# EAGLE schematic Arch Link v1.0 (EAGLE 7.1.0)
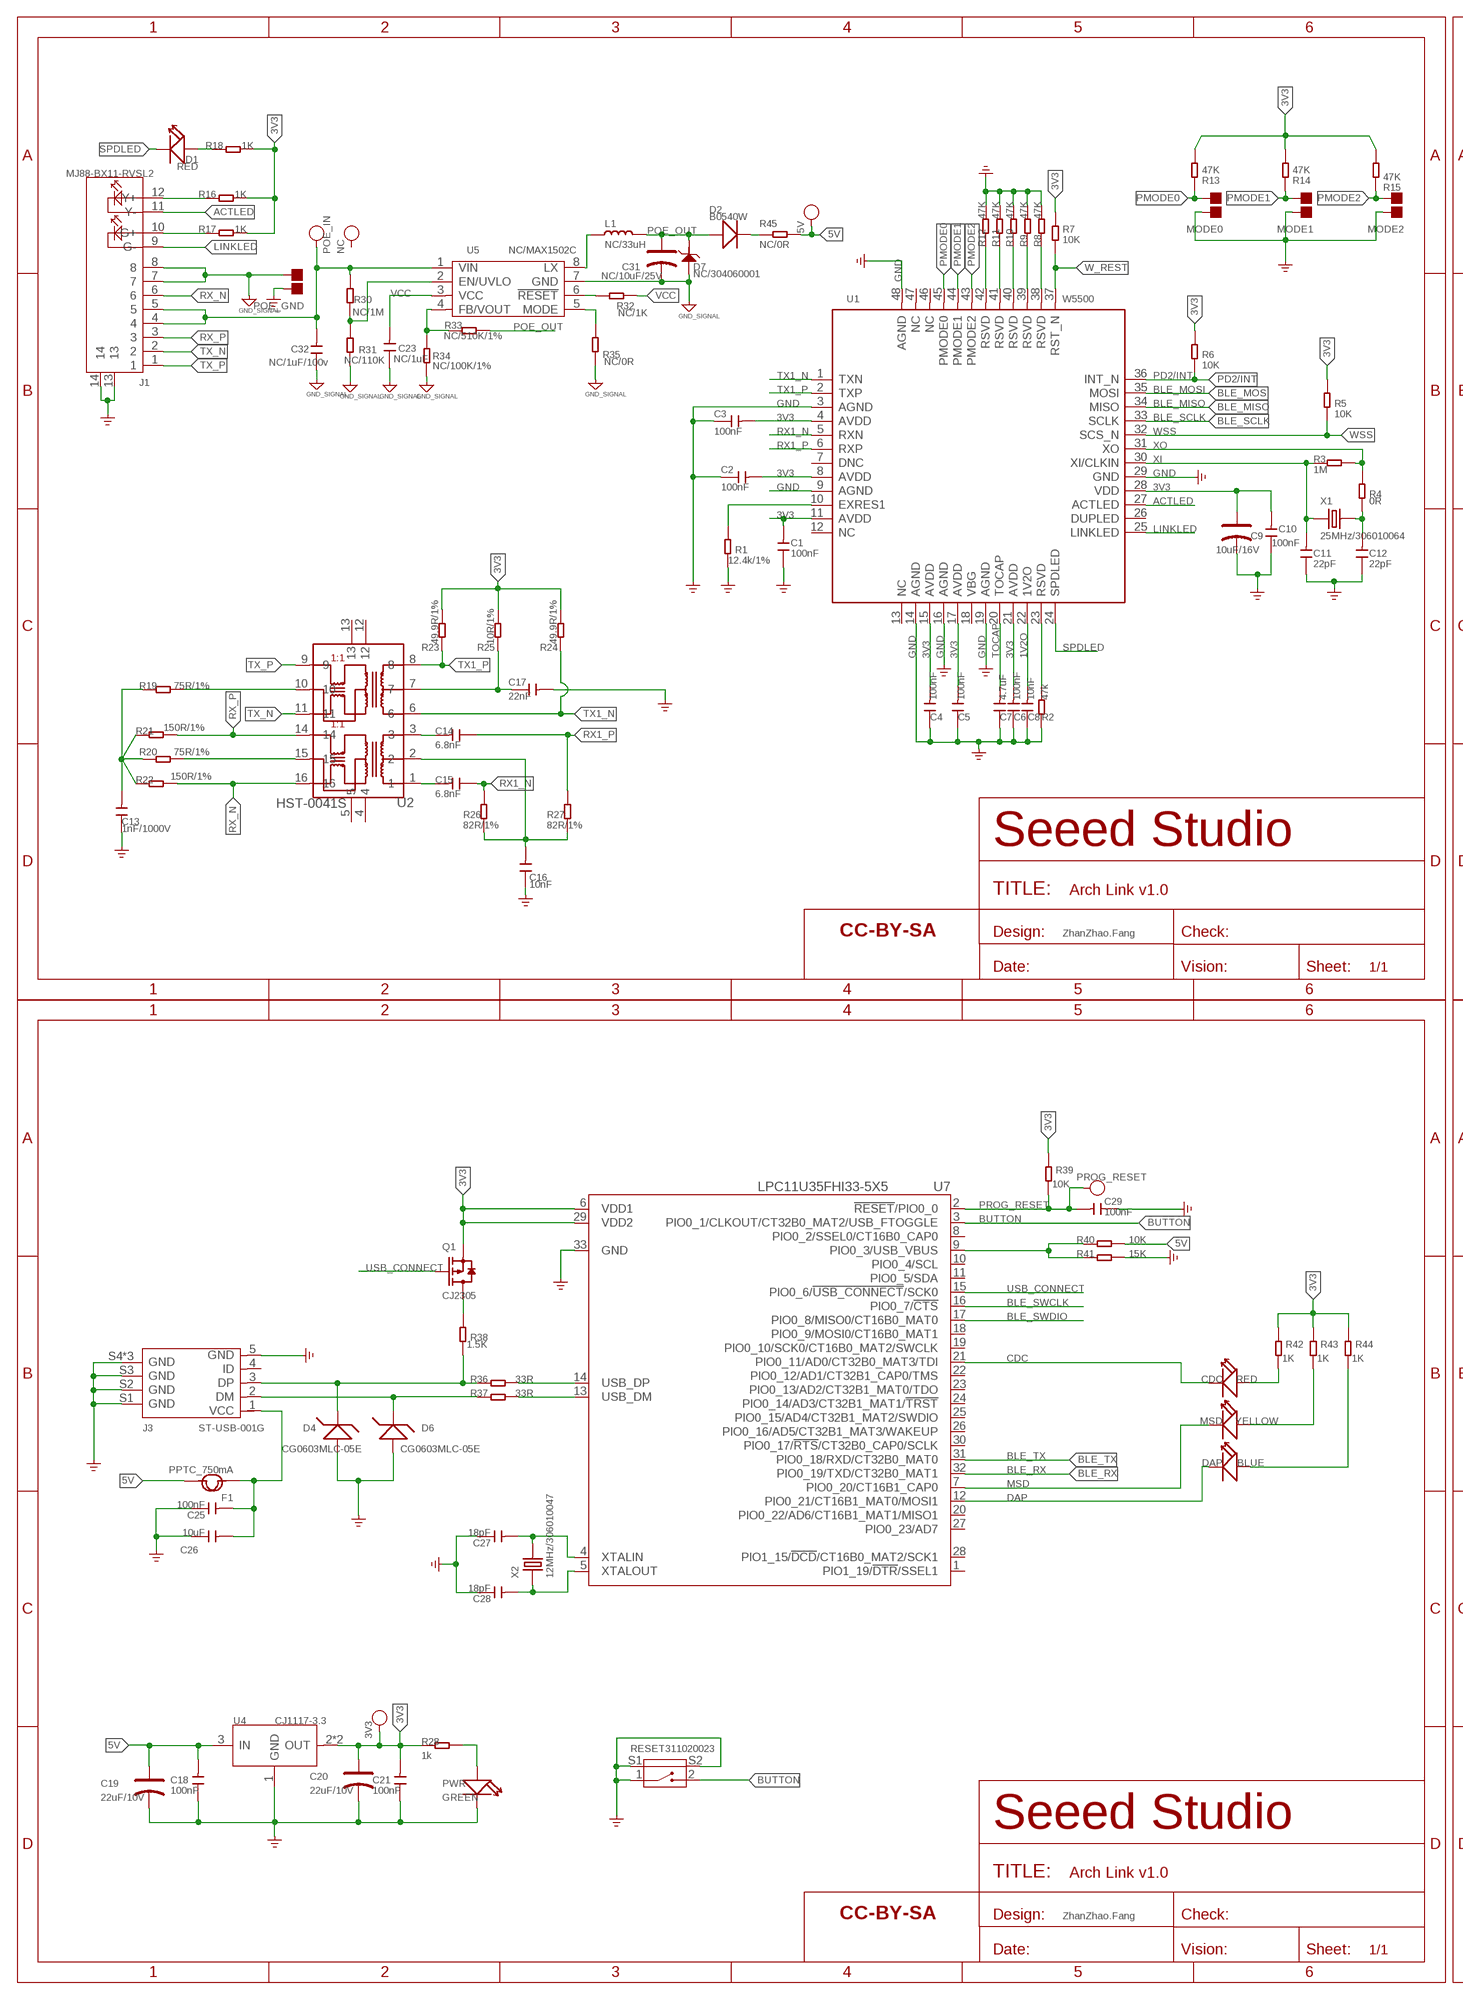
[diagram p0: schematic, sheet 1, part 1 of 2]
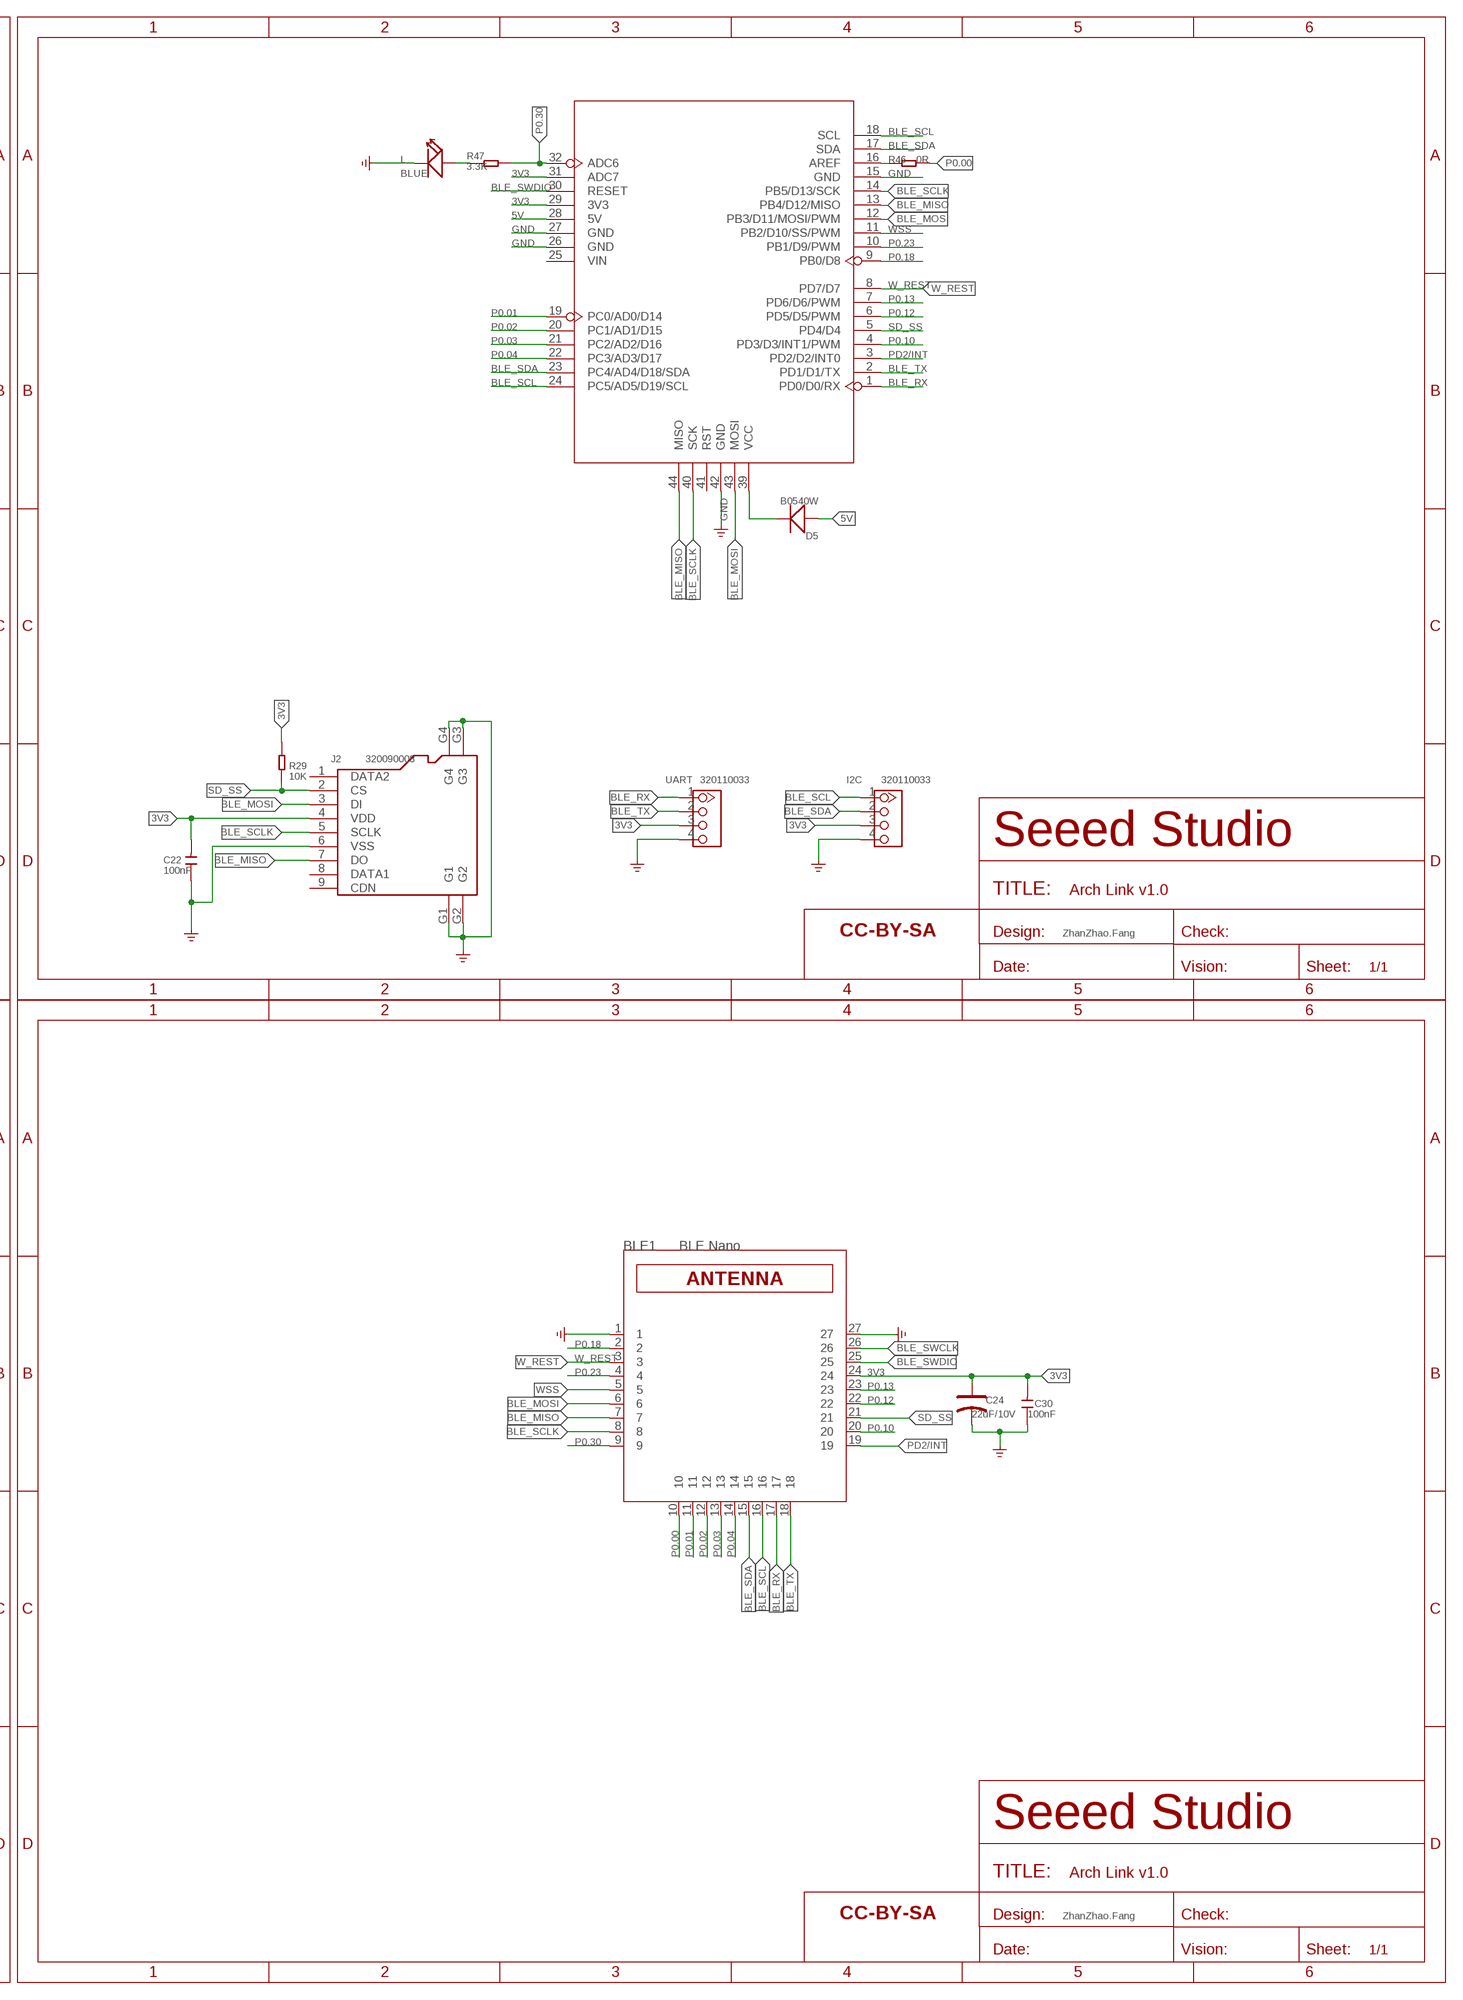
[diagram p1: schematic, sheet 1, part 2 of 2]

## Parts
3V3  TEST-POINT'4545'  [TP-D45MIL]
5V  TEST-POINT'4545'  [TP-D45MIL]
BLE1  BLE Nano  SEEED_BLE_MODULE_001'PAD'  [SEEED_BLE_MODULE_PAD]
C1  100nF  CAP-0603  [C0603]
C2  100nF  CAP-0603  [C0603]
C3  100nF  CAP-0603  [C0603]
C4  100nF  CAP-0603  [C0603]
C5  100nF  CAP-0603  [C0603]
C6  100nF  CAP-0603  [C0603]
C7  4.7uF  CAP-0603  [C0603]
C8  10nF  CAP-0603  [C0603]
C9  10uF/16V  CAP-POLAR-AVX-A  [AVX-A]
C10  100nF  CAP-0603  [C0603]
C11  22pF  CAP-0603  [C0603]
C12  22pF  CAP-0603  [C0603]
C13  1nF/1000V  CAP-1206  [C1206]
C14  6.8nF  CAP-0603  [C0603]
C15  6.8nF  CAP-0603  [C0603]
C16  10nF  CAP-0603  [C0603]
C17  22nF  CAP-0603  [C0603]
C18  100nF  CAP-0603  [C0603]
C19  22uF/10V  CAP-POLAR-AVX-B  [AVX-B]
C20  22uF/10V  CAP-POLAR-AVX-B  [AVX-B]
C21  100nF  CAP-0603  [C0603]
C22  100nF  CAP-0603  [C0603]
C23  NC/1uF  CAP-0603  [C0603]
C24  22uF/10V  CAP-POLAR-AVX-B  [AVX-B]
C25  100nF  CAP-0603  [C0603]
C26  10uF  CAP-0805  [C0805]
C27  18pF  CAP-0603  [C0603]
C28  18pF  CAP-0603  [C0603]
C29  100nF  CAP-0603  [C0603]
C30  100nF  CAP-0603  [C0603]
C31  NC/10uF/25V  CAP-POLAR-AVX-A  [AVX-A]
C32  NC/1uF/100v  CAP-1206  [C1206]
CDC  RED  LED'0603'  [LED-0603]
D1  RED  LED'0603'  [LED-0603]
D2  B0540W  DIODE'1206'  [SOD-123]
D4  CG0603MLC-05E  D-ZENER-2P'BZX584CX'  [SOD-523]
D5  B0540W  DIODE'1206'  [SOD-123]
D6  CG0603MLC-05E  D-ZENER-2P'BZX584CX'  [SOD-523]
D7  NC/304060001  D-ESD-2P'CESD5V0D1'  [SOD-123]
DAP  BLUE  LED'0603'  [LED-0603]
F1  PPTC_750mA  FUSE'1206'  [F1206]
I2C  320110033  GROVE-CONNECTOR-DIP-2.0  [HW4-2.0]
J1  MJ88-BX11-RVSL2  RJ45-MJ88-BX11-RVSL2  [RJ45-12+2P-16.3X15.4X11.5MM-IN]
J2  320090008  MICRO-SD-CARD-HOLDER-9P'MICROSD-9P'  [MICRO-SD9+4P-SMD-16.1X14.5X1.85MM]
J3  ST-USB-001G  MICRO-USB5+4P'5+4P'  [MICRO-USB5+4P-SMD-0.65-B]
L  BLUE  LED'0603'  [LED-0603]
L1  NC/33uH  INDUCTOR/FERRITE-BEAD  [INT2-SMD-4.8X4.8X3MM]
MODE0  NC  JUMPER-2P  [JUMPER-2P]
MODE1  NC  JUMPER-2P  [JUMPER-2P]
MODE2  NC  JUMPER-2P  [JUMPER-2P]
MSD  YELLOW  LED'0603'  [LED-0603]
NC  TEST-POINT'4545'  [TP-D45MIL]
POE_GND  NC  JUMPER-2P  [JUMPER-2P]
POE_IN  DNP  TEST-POINT'4545'  [TP-D45MIL]
PROG_RESET  NC  TEST-POINT'4545'  [TP-D45MIL]
PWR  GREEN  LED'0603'  [LED-0603]
Q1  CJ2305  MOSFET-P'SI2323CDS/SI2305DS<BR>'  [SOT-23]
R1  12.4k/1%  RES-0603  [R0603]
R2  47k  RES-0603  [R0603]
R3  1M  RES-0603  [R0603]
R4  0R  RES-0603  [R0603]
R5  10K  RES-0603  [R0603]
R6  10K  RES-0603  [R0603]
R7  10K  RES-0603  [R0603]
R8  47K  RES-0603  [R0603]
R9  47K  RES-0603  [R0603]
R10  47K  RES-0603  [R0603]
R11  47K  RES-0603  [R0603]
R12  47K  RES-0603  [R0603]
R13  47K  RES-0603  [R0603]
R14  47K  RES-0603  [R0603]
R15  47K  RES-0603  [R0603]
R16  1K  RES-0603  [R0603]
R17  1K  RES-0603  [R0603]
R18  1K  RES-0603  [R0603]
R19  75R/1%  RES-0603  [R0603]
R20  75R/1%  RES-0603  [R0603]
R21  150R/1%  RES-0603  [R0603]
R22  150R/1%  RES-0603  [R0603]
R23  49.9R/1%  RES-0603  [R0603]
R24  49.9R/1%  RES-0603  [R0603]
R25  10R/1%  RES-0603  [R0603]
R26  82R/1%  RES-0603  [R0603]
R27  82R/1%  RES-0603  [R0603]
R28  1k  RES-0603  [R0603]
R29  10K  RES-0603  [R0603]
R30  NC/1M  RES-0603  [R0603]
R31  NC/110K  RES-0603  [R0603]
R32  NC/1K  RES-0603  [R0603]
R33  NC/510K/1%  RES-0603  [R0603]
R34  NC/100K/1%  RES-0603  [R0603]
R35  NC/0R  RES-0603  [R0603]
R36  33R  RES-0603  [R0603]
R37  33R  RES-0603  [R0603]
R38  1.5K  RES-0603  [R0603]
R39  10K  RES-0603  [R0603]
R40  10K  RES-0603  [R0603]
R41  15K  RES-0603  [R0603]
R42  1K  RES-0603  [R0603]
R43  1K  RES-0603  [R0603]
R44  1K  RES-0603  [R0603]
R45  NC/0R  RES-0603  [R0603]
R46  0R  RES-0603  [R0603]
R47  3.3K  RES-0603  [R0603]
RESET  311020023  BUTTON-2+2P'TS-1188E'  [SW4-SMD-7.0X3.5X3.5MM-90D]
U1  W5500  INTERFACE-W5500  [LQFP48-0.5-7X7MM]
U2  HST-0041S  TRANSFORMER-HST-0041S  [SOIC16-1.27-12.7X7.0MM]
U3  DNP  SEEEDUINO_ARDUINO-44P  [SEEEDUINO-ARDUINO-DIM]
U4  CJ1117-3.3  PMIC-CJ1117S  [SOT-223]
U5  NC/MAX1502C  PMIC-MAX15062  [TDFN8-0.5-2X2MM]
U7  LPC11U35FHI33-5X5  [HVQFN33]
U$1  SEEEDSTUDIO-OPEN-SCH-FRAME  [SEEEDSTUDIO-PCB-FRAME]
U$20  SEEEDSTUDIO-OPEN-SCH-FRAME  [SEEEDSTUDIO-PCB-FRAME]
U$34  SEEEDSTUDIO-OPEN-SCH-FRAME  [SEEEDSTUDIO-PCB-FRAME]
U$38  SEEEDSTUDIO-OPEN-SCH-FRAME  [SEEEDSTUDIO-PCB-FRAME]
UART  320110033  GROVE-CONNECTOR-DIP-2.0  [HW4-2.0]
X1  25MHz/306010064  CRYSTAL'5032'  [X2-SMD-5.0X3.2X1.3MM]
X2  12MHz/306010047  CRYSTAL'5032'  [X2-SMD-5.0X3.2X1.3MM]

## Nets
1: R2.2 U1.23(RSVD)
1V2O: C8.2 U1.22(1V2O)
2: R8.2 U1.38(RSVD)
3: R9.2 U1.39(RSVD)
3V3: 3V3.T BLE1.24 C1.2 C2.2 C3.2 C4.2 C5.2 C6.2 C9.+ C10.2 C20.+ C21.2 C22.2 C24.+ C30.2 I2C.3 J2.4(VDD) Q1.2(S) R5.1 R6.1 R7.1 R13.1 R14.1 R15.1 R16.2 R17.2 R18.2 R23.1 R24.1 R25.1 R28.2 R29.1 R39.2 R42.2 R43.2 R44.2 U1.4(AVDD) U1.8(AVDD) U1.11(AVDD) U1.15(AVDD) U1.17(AVDD) U1.21(AVDD) U1.28(VDD) U3.29(3V3) U3.31(ADC7) U4.2(OUT) U4.TER(OUT) U7.6(VDD1) U7.29(VDD2) UART.3
4: R10.2 U1.40(RSVD)
5: R11.2 U1.41(RSVD)
5V: 5V.T C18.2 C19.+ D5.+ F1.2 R40.1 R45.2 U3.28(5V) U4.3(IN)
6: R12.2 U1.42(RSVD)
ACTLED: J1.11(Y-) U1.27(ACTLED)
AGND: C23.1 C31.- C32.1 D7.+ J1.7 J1.8 POE_GND.1 R31.1 R34.2 R35.2 U5.7(GND) ; supply symbol labelled GND_SIGNAL
BLE_MISO: BLE1.7 J2.7(DO) U1.34(MISO) U3.13(PB4/D12/MISO) U3.44(MISO)
BLE_MOSI: BLE1.6 J2.3(DI) U1.35(MOSI) U3.12(PB3/D11/MOSI/PWM) U3.43(MOSI)
BLE_RX: BLE1.17 U3.1(PD0/D0/RX) U7.32(PIO0_19/TXD/CT32B0_MAT1) UART.1
BLE_SCL: BLE1.16 I2C.1 U3.18(SCL) U3.24(PC5/AD5/D19/SCL)
BLE_SCLK: BLE1.8 J2.5(SCLK) U1.33(SCLK) U3.14(PB5/D13/SCK) U3.40(SCK)
BLE_SDA: BLE1.15 I2C.2 U3.17(SDA) U3.23(PC4/AD4/D18/SDA)
BLE_SWCLK: BLE1.26 U7.16(PIO0_7/!CTS!)
BLE_SWDIO: BLE1.25 U3.30(RESET) U7.17(PIO0_8/MISO0/CT16B0_MAT0)
BLE_TX: BLE1.18 U3.2(PD1/D1/TX) U7.31(PIO0_18/RXD/CT32B0_MAT0) UART.2
BUTTON: RESET.2 U7.3(PIO0_1/CLKOUT/CT32B0_MAT2/USB_FTOGGLE)
CDC: CDC.- U7.21(PIO0_11/AD0/CT32B0_MAT3/TDI)
DAP: DAP.- U7.12(PIO0_21/CT16B1_MAT0/MOSI1)
GND: BLE1.1 BLE1.27 C1.1 C2.1 C3.1 C4.1 C5.1 C6.1 C7.1 C8.1 C9.- C10.1 C11.1 C12.1 C13.1 C16.1 C17.2 C18.1 C19.- C20.- C21.1 C22.1 C24.- C25.1 C26.1 C27.1 C28.1 C29.1 C30.1 D4.+ D6.+ I2C.4 J1.13 J1.14 J2.6(VSS) J2.G1 J2.G2 J2.G3 J2.G4 J3.5(GND) J3.S1(GND) J3.S2(GND) J3.S3(GND) J3.S4(GND) J3.S5(GND) J3.S6(GND) L.- MODE0.2 MODE1.2 MODE2.2 POE_GND.2 PWR.- R1.1 R2.1 R8.1 R9.1 R10.1 R11.1 R12.1 R41.1 RESET.1 RESET.S1 RESET.S2 U1.3(AGND) U1.9(AGND) U1.14(AGND) U1.16(AGND) U1.19(AGND) U1.29(GND) U1.48(AGND) U3.15(GND) U3.26(GND) U3.27(GND) U3.42(GND) U4.1(GND) U7.33(GND) UART.4 ; supply symbol labelled GND_POWER
LINKLED: J1.9(G-) U1.25(LINKLED)
MSD: MSD.- U7.7(PIO0_20/CT16B1_CAP0)
N$1: R1.2 U1.10(EXRES1)
N$2: J1.12(Y+) R16.1
N$4: J1.10(G+) R17.1
N$5: C12.2 R4.2 X1.2
N$6: D1.+ R18.1
N$8: C13.2 R19.2 R20.2 R21.2 R22.1
N$9: C15.2 U2.1
N$10: C32.2 J1.4 J1.5 POE_IN.T R30.2 U5.1(VIN)
N$11: R19.1 U2.10
N$12: R36.2 U7.14(USB_DP)
N$13: C14.2 U2.3
N$14: CDC.+ R42.1
N$15: C16.2 R26.2 R27.2 U2.2
N$16: R37.2 U7.13(USB_DM)
N$17: R20.1 U2.15
N$18: R33.2 R34.1 U5.4(FB/VOUT)
N$19: R30.1 R31.2 U5.2(EN/UVLO)
N$20: C17.1 R25.2 U2.7
N$21: D4.- J3.3(DP) R36.1 R38.1
N$22: R46.2 U3.16(AREF)
N$23: D6.- J3.2(DM) R37.1
N$24: PWR.+ R28.1
N$26: C25.2 C26.2 F1.1 J3.1(VCC)
N$28: C27.2 U7.4(XTALIN) X2.2
N$29: C28.2 U7.5(XTALOUT) X2.1
N$30: R32.2 U5.6(!RESET)
N$31: R40.2 R41.2 U7.9(PIO0_3/USB_VBUS)
N$32: R35.1 U5.5(MODE)
N$33: MSD.+ R43.1
N$34: DAP.+ R44.1
N$35: L.+ R47.1
N$36: Q1.3(D) R38.2
N$37: L1.1 U5.8(LX)
N$39: D2.- R45.1
P0.00: BLE1.10 R46.1
P0.01: BLE1.11 U3.19(PC0/AD0/D14)
P0.02: BLE1.12 U3.20(PC1/AD1/D15)
P0.03: BLE1.13 U3.21(PC2/AD2/D16)
P0.04: BLE1.14 U3.22(PC3/AD3/D17)
P0.10: BLE1.20 U3.4(PD3/D3/INT1/PWM)
P0.12: BLE1.22 U3.6(PD5/D5/PWM)
P0.13: BLE1.23 U3.7(PD6/D6/PWM)
P0.18: BLE1.2 U3.9(PB0/D8)
P0.23: BLE1.4 U3.10(PB1/D9/PWM)
P0.30: BLE1.9 R47.2 U3.32(ADC6)
PD2/INT: BLE1.19 R6.2 U1.36(INT_N) U3.3(PD2/D2/INT0)
PMODE0: MODE0.1 R13.2 U1.45(PMODE0)
PMODE1: MODE1.1 R14.2 U1.44(PMODE1)
PMODE2: MODE2.1 R15.2 U1.43(PMODE2)
POE_OUT: C31.+ D2.+ D7.- L1.2 R33.1
PROG_RESET: C29.2 PROG_RESET.T R39.1 U7.2(!RESET!/PIO0_0)
RX1_N: C15.1 R26.1 U1.5(RXN)
RX1_P: C14.1 R27.1 U1.6(RXP)
RX_N: J1.6 R22.2 U2.16
RX_P: J1.3 R21.1 U2.14
SD_SS: BLE1.21 J2.2(CS) R29.2 U3.5(PD4/D4)
SPDLED: D1.- U1.24(SPDLED)
TOCAP: C7.2 U1.20(TOCAP)
TX1_N: R24.2 U1.1(TXN) U2.6
TX1_P: R23.2 U1.2(TXP) U2.8
TX_N: J1.2 U2.11
TX_P: J1.1 U2.9
USB_CONNECT: Q1.1(G) U7.15(PIO0_6/!USB_CONNECT!/SCK0)
VCC: C23.2 R32.1 U5.3(VCC)
VCC1: D5.- U3.39(VCC)
W_REST: BLE1.3 R7.2 U1.37(RST_N) U3.8(PD7/D7)
WSS: BLE1.5 R5.2 U1.32(SCS_N) U3.11(PB2/D10/SS/PWM)
XI: C11.2 R3.2 U1.30(XI/CLKIN) X1.1
XO: R3.1 R4.1 U1.31(XO)
Unconnected: J2.1(DATA2) J2.8(DATA1) J2.9(CDN) J3.4(ID) NC.T U1.7(DNC) U1.12(NC) U1.13(NC) U1.18(VBG) U1.26(DUPLED) U1.46(NC) U1.47(NC) U2.4 U2.5 U2.12 U2.13 U3.25(VIN) U3.41(RST) U7.1(PIO1_19/!DTR!/SSEL1) U7.8(PIO0_2/SSEL0/CT16B0_CAP0) U7.10(PIO0_4/SCL) U7.11(PIO0_5/SDA) U7.18(PIO0_9/MOSI0/CT16B0_MAT1) U7.19(PIO0_10/SCK0/CT16B0_MAT2/SWCLK) U7.20(PIO0_22/AD6/CT16B1_MAT1/MISO1) U7.22(PIO0_12/AD1/CT32B1_CAP0/TMS) U7.23(PIO0_13/AD2/CT32B1_MAT0/TDO) U7.24(PIO0_14/AD3/CT32B1_MAT1/!TRST!) U7.25(PIO0_15/AD4/CT32B1_MAT2/SWDIO) U7.26(PIO0_16/AD5/CT32B1_MAT3/WAKEUP) U7.27(PIO0_23/AD7) U7.28(PIO1_15/!DCD!/CT16B0_MAT2/SCK1) U7.30(PIO0_17/!RTS!/CT32B0_CAP0/SCLK)

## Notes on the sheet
- ZhanZhao.Fang | ZhanZhao.Fang
- ZhanZhao.Fang | ZhanZhao.Fang

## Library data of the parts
3V3 5V NC POE_IN PROG_RESET = Discrete-new:TEST-POINT; PARTNO: DNP
BLE1 = AMLib_New:SEEED_BLE_MODULE_001
C1-C8 C10-C18 C21-C23 C25-C30 C32 = Discrete-new:CAP: Ceramic Capacitors
C9 C19 C20 C24 C31 = Discrete-new:CAP-POLAR: Electrolytic Capacitors,Tantalum Capacitors and Super Capacitors
CDC D1 DAP L MSD PWR = Discrete-new:LED
D2 D5 = Discrete-new:DIODE*
D4 D6 = Discrete-new:D-ZENER-2P: SOD-123:304030008;SOT-23:304030000
D7 = Discrete-new:D-ESD-2P: SOD-923:304060009;SOD-123:304060001
F1 = Discrete-new:FUSE
I2C UART = Connector-new:GROVE-CONNECTOR-DIP: 4P-2.0:320110033;4P-2.0-90D:320110034
J1 = Connector-new:RJ45-MJ88-BX11-RVSL2: 320140004
J2 = Connector-new:MICRO-SD-CARD-HOLDER-9P: 320090000
J3 = Connector-new:MICRO-USB5+4P: 5+4P-SMD-0.65-B:320010000;5+2P-SMD-0.65-AB:340032001
L1 = Discrete-new:INDUCTOR/FERRITE-BEAD
MODE0 MODE1 MODE2 POE_GND = Discrete-new:JUMPER-2P; PARTNO: DNP
Q1 = Discrete-new:MOSFET-P
R1-R47 = Discrete-new:RES
RESET = Discrete-new:BUTTON-2+2P: SW4-SMD-4.5X3.8X1.8MM-90D:311020035;SW4-SMD-7.0X3.5X3.5MM-90D:311020023
U1 = IC-new:INTERFACE-W5500: 310070032
U2 = template:TRANSFORMER-HST-0041S: 10/100BASE-T Single Port Surface Mount Magnetics With Various Turns Ratios
U3 = Antenna:SEEEDUINO_ARDUINO-44P
U4 = IC-new:PMIC-CJ*1117: Low Drop Fixed And Adjustable Positive Voltage Regulators http://www.datasheetcatalog.org/datasheet/SGSThomsonMicroelectronics/mXuqtqv.pdf
U5 = template:PMIC-MAX15062
U7 = AMLib_New:LPC11U35FHI33
U$1 U$20 U$34 U$38 = moudle-new:SEEEDSTUDIO-OPEN-SCH-FRAME
X1 X2 = Discrete-new:CRYSTAL

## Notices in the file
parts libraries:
moudle-new: This work is licensed under the Creative Commons Attribution 4.0 International License.
To view a copy of this license,visit:
http://creativecommons.org/licenses/by-sa/4.0
moudle-new: CC-BY-SA
